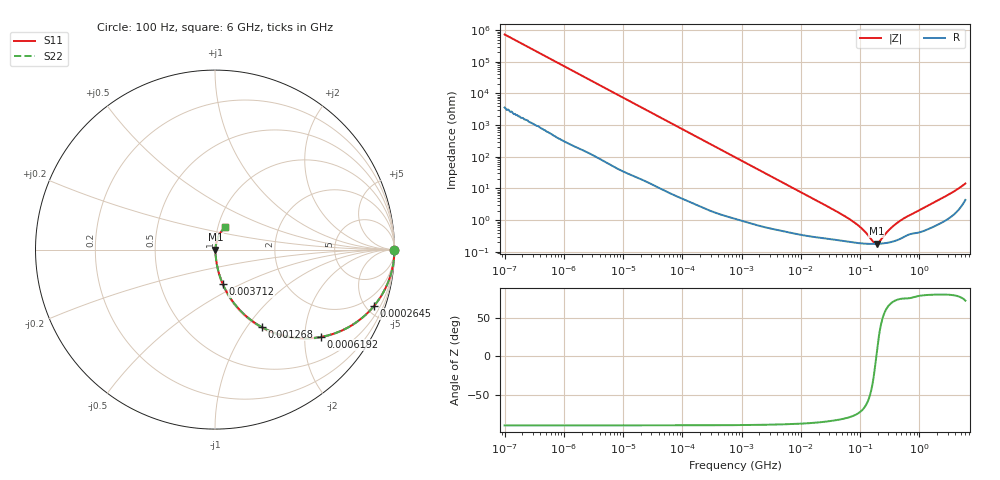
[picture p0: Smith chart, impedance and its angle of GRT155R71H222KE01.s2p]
!Murata Part Number: GRT155R71H222KE01
!These Parameters are Measured in Series Mode Connection
!Data Generated on Jun 19, 2026
!  o--ll--o
!Port1  Port2
!  o------o
!Operation Temp=25[degC], DC Bias Voltage=0[V]
!Freq. Start=100[Hz] Stop=6[GHz] 401[Steps]
# Hz S RI R 50
!Freq.(Hz) S11(Real) S11(Imag) S21(Real) S21(Imag) S12(Real) S12(Imag) S22(Real) S22(Imag)
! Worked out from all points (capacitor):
!   401 points, 100 Hz to 6 GHz, reference 50 ohm
!   read as one part in series: C = 2.19 nF near 109 Hz
!   lowest |Z| = 179 mohm at 190.9 MHz (marker M1)
!   series resonance near 188.1 MHz, so ESL is about 330 pH
!   S11 on the Smith chart (normalised r, x): 100 Hz: open; 264.5 kHz: 1.04, -5.63; 619.2 kHz: 1.02, -2.41; 1.268 MHz: 1.02, -1.18; 3.712 MHz: 1.01, -0.41; 6 GHz: 1.09, +0.27
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100  1 -0.000138  7e-07 0.000138  7e-07 0.000138  1 -0.000138
2008  1 -0.00274  2e-05 0.00274  2e-05 0.00274  1 -0.00274
40335  0.9967 -0.0543  0.00327 0.0543  0.00327 0.0543  0.9967 -0.0543
108014  0.9784 -0.1423  0.0216 0.1423  0.0216 0.1423  0.9784 -0.1423
264476  0.8861 -0.3138  0.1139 0.3138  0.1139 0.3138  0.8861 -0.3138
395726  0.7784 -0.4111  0.2216 0.4111  0.2216 0.4111  0.7784 -0.4111
619225  0.592 -0.4863  0.408 0.4863  0.408 0.4863  0.592 -0.4863
774597  0.4828 -0.494  0.5172 0.494  0.5172 0.494  0.4828 -0.494
1267578  0.2625 -0.4329  0.7375 0.4329  0.7375 0.4329  0.2625 -0.4329
2074311  0.1208 -0.317  0.8792 0.317  0.8792 0.317  0.1208 -0.317
3712478  0.0443 -0.1937  0.9557 0.1937  0.9557 0.1937  0.0443 -0.1937
7266822  0.0146 -0.1028  0.9854 0.1028  0.9854 0.1028  0.0146 -0.1028
1.555665e7  0.00538 -0.0488  0.9946 0.0488  0.9946 0.0488  0.00538 -0.0488
7.455971e7  0.00207 -0.00907  0.9979 0.00907  0.9979 0.00907  0.00207 -0.00907
1.115611e8  0.00185 -0.00471  0.9982 0.00471  0.9982 0.00471  0.00185 -0.00471
1.669249e8  0.00177 -0.00104  0.9982 0.00104  0.9982 0.00104  0.00177 -0.00104
1.909225e8  0.00178 0.000133  0.9982 -0.000133  0.9982 -0.000133  0.00178 0.000133
2.183701e8  0.00181 0.00131  0.9982 -0.00131  0.9982 -0.00131  0.00181 0.00131
3.124326e8  0.002 0.00461  0.998 -0.00461  0.998 -0.00461  0.002 0.00461
5.59173e8  0.00311 0.0112  0.9969 -0.0112  0.9969 -0.0112  0.00311 0.0112
2.34314e9  0.0103 0.0463  0.9897 -0.0463  0.9897 -0.0463  0.0103 0.0463
6e9  0.0578 0.1233  0.9422 -0.1233  0.9422 -0.1233  0.0578 0.1233
